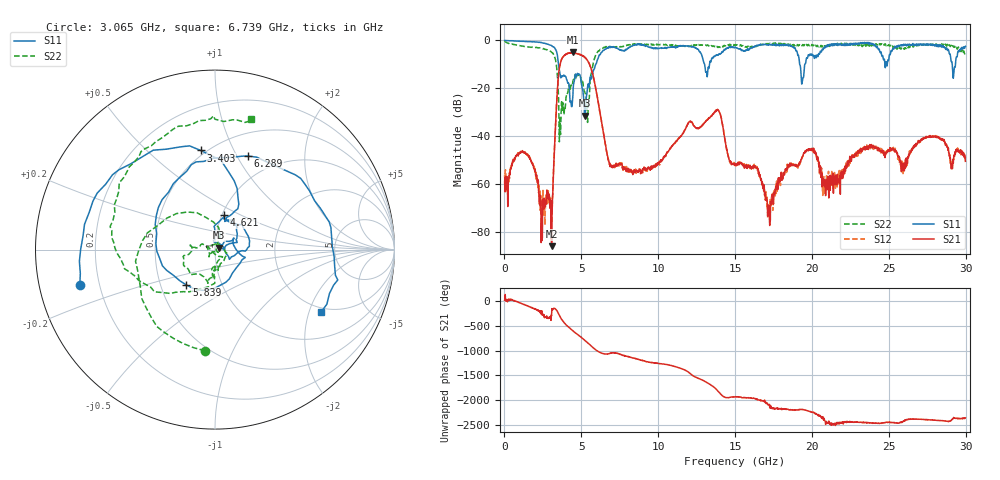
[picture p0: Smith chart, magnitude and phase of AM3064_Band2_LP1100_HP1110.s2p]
# Hz S DB R 50.0
!freq dBS11 angS11 dBS21 angS21 dBS12 angS12 dBS22 angS22
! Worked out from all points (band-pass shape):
!   1600 points, 10 MHz to 29.98 GHz, reference 50 ohm
!   highest |S21| = -5.06 dB at 4.434 GHz (marker M1); lowest = -85.7 dB at 3.065 GHz (marker M2)
!   |S21| within 3 dB of the highest: 3.705 GHz to 5.357 GHz (1.652 GHz wide, 36.5 % of centre)
!   lowest |S11| = -31.4 dB at 5.221 GHz (marker M3), VSWR 1.06, Z = 52.5 + j1.22 ohm
!   |S11| at or under -10 dB: 3.516 GHz to 5.939 GHz (2.423 GHz wide, 51.3 % of centre); 13.02 GHz to 13.34 GHz (321.1 MHz wide, 2.44 % of centre); 19.2 GHz to 19.54 GHz (333.8 MHz wide, 1.72 % of centre)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
!   |S22| runs from -42.3 to -0.3 dB; largest |S21 - S12| = 0.018
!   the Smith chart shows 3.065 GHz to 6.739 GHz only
!   S11 on the Smith chart (normalised r, x): 3.065 GHz: 0.13, -0.13; 3.403 GHz: 0.47, +0.75; 4.621 GHz: 1.03, +0.41; 5.839 GHz: 0.68, -0.28; 6.289 GHz: 0.74, +1.11; 6.739 GHz: 1.85, -2.42
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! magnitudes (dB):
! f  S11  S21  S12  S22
! 10 MHz  0.0  -59.3  -56.2  -0.3
! 1.247 GHz  -0.5  -46.5  -46.6  -2.5
! 2.409 GHz  -0.9  -77.1  -70.4  -3.3
! 3.065 GHz  -2.2  -85.7  -75.5  -4.9
! 3.403 GHz  -5.1  -25.1  -25.2  -11.7
! 3.703 GHz  -15.2  -8.1  -8.2  -26.4
! 4.434 GHz  -24.9  -5.1  -5.2  -17.9
! 4.621 GHz  -14.0  -5.4  -5.4  -14.8
! 5.015 GHz  -18.4  -6.2  -6.2  -17.8
! 5.221 GHz  -31.4  -7.0  -7.0  -21.4
! 5.839 GHz  -11.9  -16.9  -16.8  -7.7
! 6.289 GHz  -5.1  -33.0  -32.7  -3.6
! 6.739 GHz  -3.3  -49.3  -49.6  -2.4
! 10 GHz  -3.4  -50.9  -51.5  -1.8
! 13.82 GHz  -6.0  -28.9  -29.0  -2.5
! 15 GHz  -2.8  -51.4  -52.0  -1.8
! 16.39 GHz  -2.2  -53.1  -53.5  -2.5
! 17.25 GHz  -1.7  -77.1  -71.8  -1.2
! 19.99 GHz  -5.7  -45.1  -45.1  -1.7
! 21.04 GHz  -2.0  -56.6  -59.3  -2.1
! 25 GHz  -8.0  -45.7  -46.1  -1.8
! 29.98 GHz  -2.5  -50.4  -48.6  -4.7
